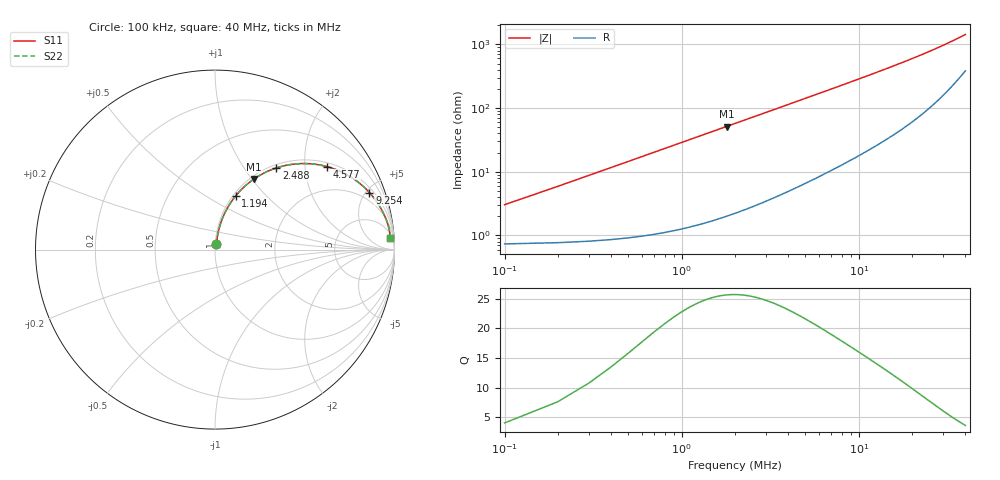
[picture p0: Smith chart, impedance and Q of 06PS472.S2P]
! Coilcraft 0603PS-472 Power Chip Inductor
! 19 February 2003
# MHZ S MA R 50
!Freq  MagS11  AngS11  MagS21  AngS21  MagS12  AngS12  MagS22  AngS22
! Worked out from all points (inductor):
!   403 points, 100 kHz to 40 MHz, reference 50 ohm
!   read as one part in series: L = 4.63 uH near 299 kHz
!   highest Q = 25.6 at 1.792 MHz (marker M1), where L = 4.56 uH
!   S11 on the Smith chart (normalised r, x): 100 kHz: 1.01, +0.06; 1.194 MHz: 1.03, +0.69; 2.488 MHz: 1.06, +1.42; 4.577 MHz: 1.12, +2.60; 9.254 MHz: 1.32, +5.27; 40 MHz: 9, +28
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0.1  0.03019 74.3  0.9923 -1.7  0.9923 -1.7  0.03019 74.3
0.1995  0.05843 79.2  0.9907 -3.3  0.9907 -3.3  0.05843 79.2
0.299  0.08661 79.7  0.9882 -4.9  0.9882 -4.9  0.08661 79.7
0.3985  0.1145 79.2  0.985 -6.6  0.985 -6.6  0.1145 79.2
0.498  0.1421 78.2  0.9809 -8.2  0.9809 -8.2  0.1421 78.2
0.5975  0.1692 77.0  0.9761 -9.7  0.9761 -9.7  0.1692 77.0
0.697  0.1959 75.8  0.9706 -11.3  0.9706 -11.3  0.1959 75.8
0.896  0.2478 73.0  0.9576 -14.3  0.9576 -14.3  0.2478 73.0
1.1945  0.3211 68.9  0.9338 -18.7  0.9338 -18.7  0.3211 68.9
1.493  0.3885 64.9  0.9062 -22.8  0.9062 -22.8  0.3885 64.9
1.7915  0.4497 61.1  0.8758 -26.7  0.8758 -26.7  0.4497 61.1
2.488  0.5689 53.1  0.8003 -34.6  0.8003 -34.6  0.5689 53.1
3.3835  0.6802 44.8  0.7054 -42.8  0.7054 -42.8  0.6802 44.8
4.5775  0.7764 36.6  0.5963 -50.9  0.5963 -50.9  0.7764 36.6
5.5725  0.8279 31.5  0.5225 -55.8  0.5225 -55.8  0.8279 31.5
6.7665  0.8691 26.8  0.4516 -60.2  0.4516 -60.2  0.8691 26.8
9.254  0.9172 20.3  0.3473 -66.3  0.3473 -66.3  0.9172 20.3
13.433  0.9515 14.2  0.2452 -71.6  0.2452 -71.6  0.9515 14.2
20.0995  0.9706 9.2  0.1616 -74.9  0.1616 -74.9  0.9706 9.2
26.766  0.9771 6.6  0.1163 -75.3  0.1163 -75.3  0.9771 6.6
33.4325  0.9792 4.9  0.08776 -73.9  0.08776 -73.9  0.9792 4.9
40  0.9794 3.8  0.06851 -70.6  0.06851 -70.6  0.9794 3.8
